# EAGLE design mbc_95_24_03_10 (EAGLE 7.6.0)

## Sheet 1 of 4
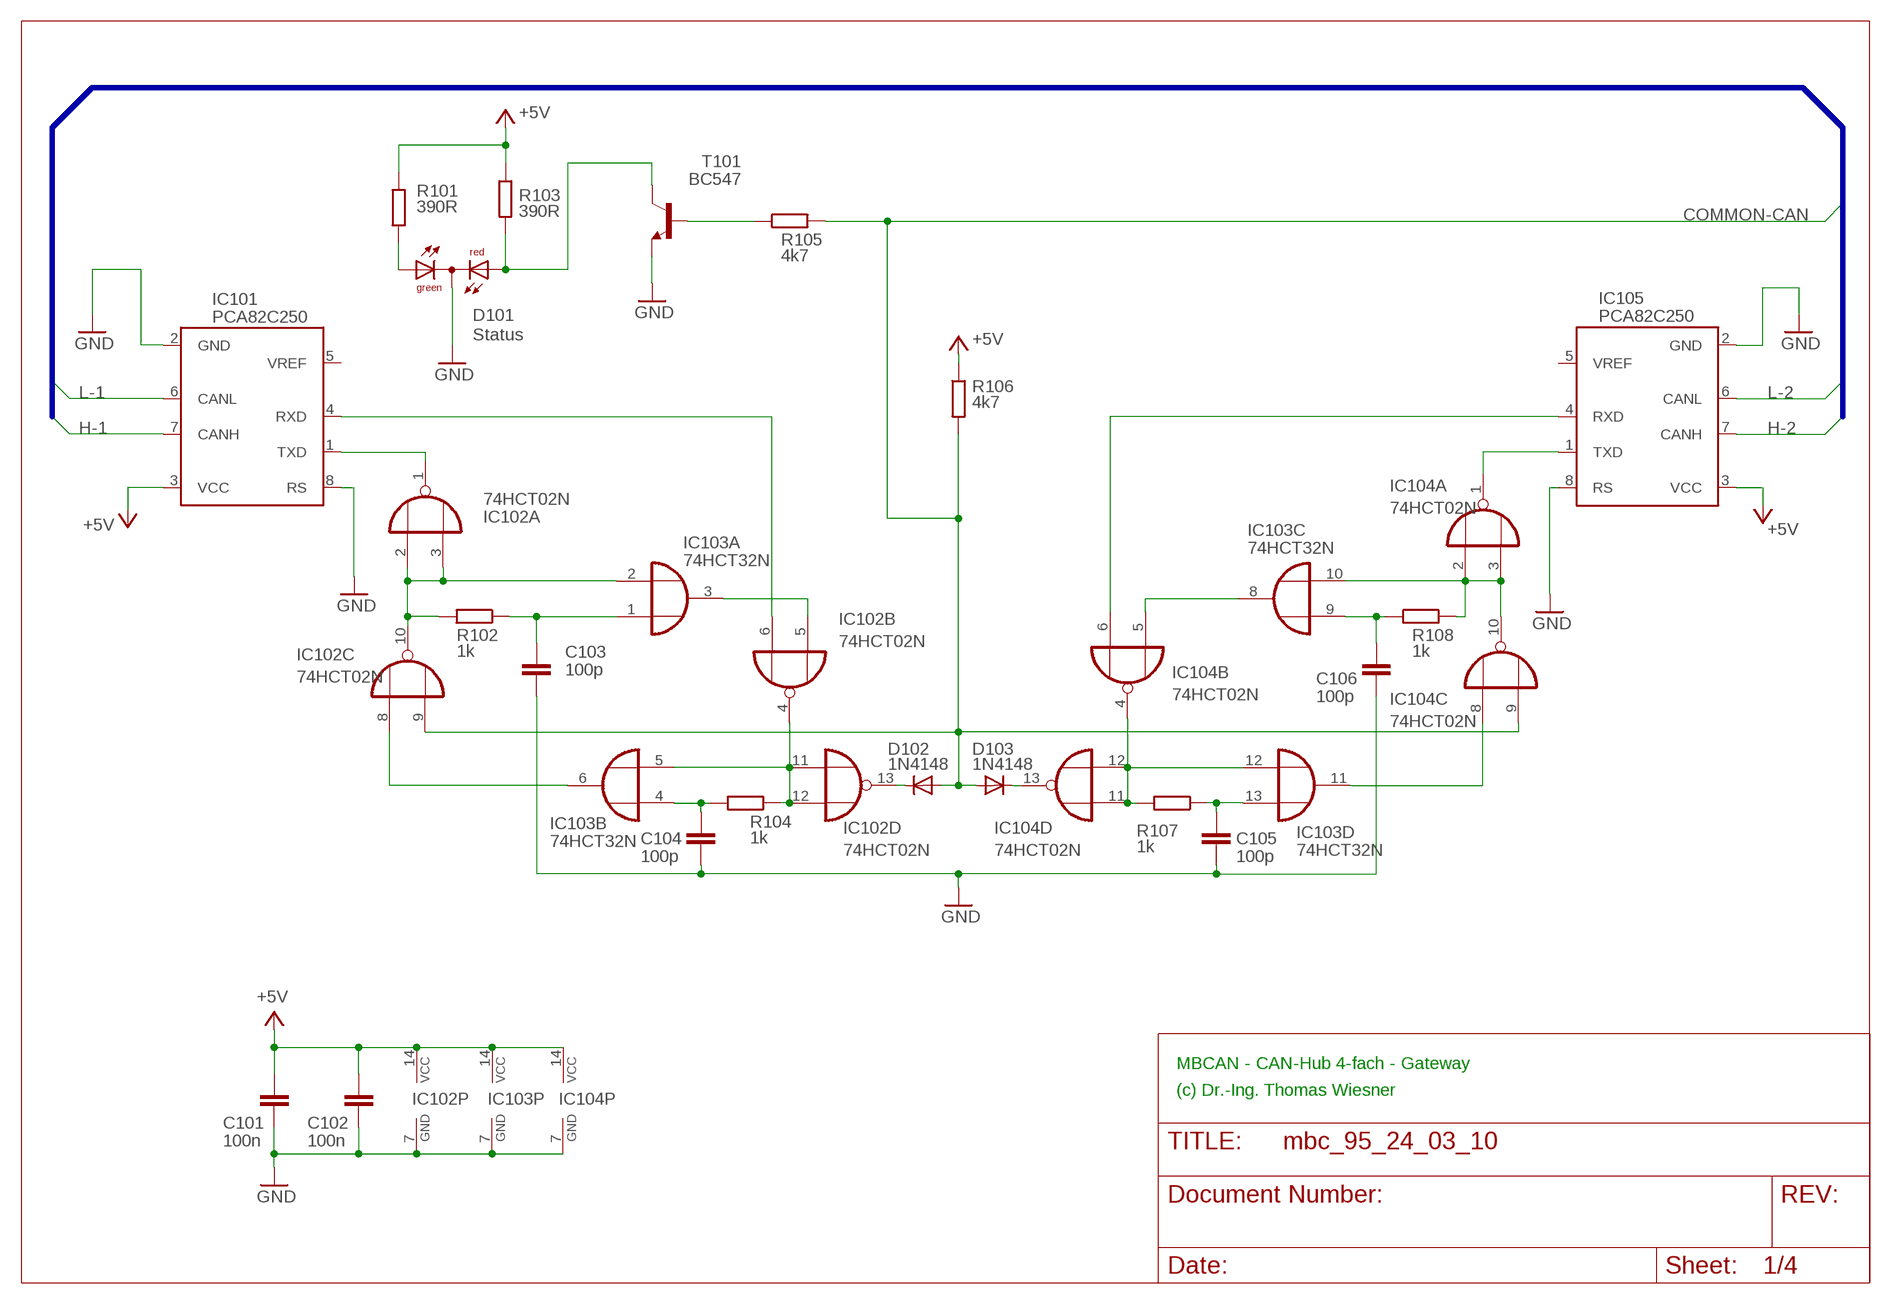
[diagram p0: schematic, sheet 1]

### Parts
C101  100n  C-EU025-025X050  [C025-025X050]
C102  100n  C-EU025-025X050  [C025-025X050]
C103  100p  C-EU025-025X050  [C025-025X050]
C104  100p  C-EU025-025X050  [C025-025X050]
C105  100p  C-EU025-025X050  [C025-025X050]
C106  100p  C-EU025-025X050  [C025-025X050]
D101  Status  DUOLED5MM  [DUOLED5MM]
D102  1N4148  1N4148DO35-10  [DO35-10]
D103  1N4148  1N4148DO35-10  [DO35-10]
IC101  PCA82C250  [DIL08]
IC102  74HCT02N  74HC02N  [DIL14]
IC103  74HCT32N  74HC32N  [DIL14]
IC104  74HCT02N  74HC02N  [DIL14]
IC105  PCA82C250  [DIL08]
R101  390R  R-EU_0207/10  [0207/10]
R102  1k  R-EU_0207/10  [0207/10]
R103  390R  R-EU_0207/10  [0207/10]
R104  1k  R-EU_0207/10  [0207/10]
R105  4k7  R-EU_0207/10  [0207/10]
R106  4k7  R-EU_0207/10  [0207/10]
R107  1k  R-EU_0207/10  [0207/10]
R108  1k  R-EU_0207/10  [0207/10]
T101  BC547  -NPN-TO92  [TO92]

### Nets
+5V: C101.2 C102.2 IC101.3(VCC) IC102.14(P:VCC) IC103.14(P:VCC) IC104.14(P:VCC) IC105.3(VCC) R101.1 R103.1 R106.1 ; also sheet 2,3,4
COMMON-CAN: D102.A D103.A IC102.9(C:I1) IC104.9(C:I1) R105.2 R106.2 ; also sheet 2,3
GND: C101.1 C102.1 C103.2 C104.2 C105.2 C106.2 D101.K(C) IC101.2(GND) IC101.8(RS) IC102.7(P:GND) IC103.7(P:GND) IC104.7(P:GND) IC105.2(GND) IC105.8(RS) T101.1(E) ; also sheet 2,3,4
H-1: IC101.7(CANH) ; also sheet 4
H-2: IC105.7(CANH) ; also sheet 4
L-1: IC101.6(CANL) ; also sheet 4
L-2: IC105.6(CANL) ; also sheet 4
N$1: IC102.2(A:I0) IC102.3(A:I1) IC102.10(C:O) IC103.2(A:I1) R102.2
N$2: R105.1 T101.2(B)
N$6: IC104.6(B:I1) IC105.4(RXD)
N$9: D101.AR R103.2 T101.3(C)
N$11: C103.1 IC103.1(A:I0) R102.1
N$13: D101.AG R101.2
N$14: IC101.1(TXD) IC102.1(A:O)
N$15: IC102.5(B:I0) IC103.3(A:O)
N$16: IC104.1(A:O) IC105.1(TXD)
N$17: IC102.8(C:I0) IC103.6(B:O)
N$18: C104.1 IC103.4(B:I0) R104.2
N$19: IC102.4(B:O) IC102.11(D:I0) IC102.12(D:I1) IC103.5(B:I1) R104.1
N$21: D102.C IC102.13(D:O)
N$25: IC101.4(RXD) IC102.6(B:I1)
N$27: D103.C IC104.13(D:O)
N$29: IC103.12(D:I0) IC104.4(B:O) IC104.11(D:I0) IC104.12(D:I1) R107.2
N$31: C105.1 IC103.13(D:I1) R107.1
N$33: IC103.11(D:O) IC104.8(C:I0)
N$34: IC103.10(C:I1) IC104.2(A:I0) IC104.3(A:I1) IC104.10(C:O) R108.1
N$36: C106.1 IC103.9(C:I0) R108.2
N$37: IC103.8(C:O) IC104.5(B:I0)
Unconnected: IC101.5(VREF) IC105.5(VREF)

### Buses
B$2

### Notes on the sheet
- MBCAN - CAN-Hub 4-fach - Gateway
- (c) Dr.-Ing. Thomas Wiesner

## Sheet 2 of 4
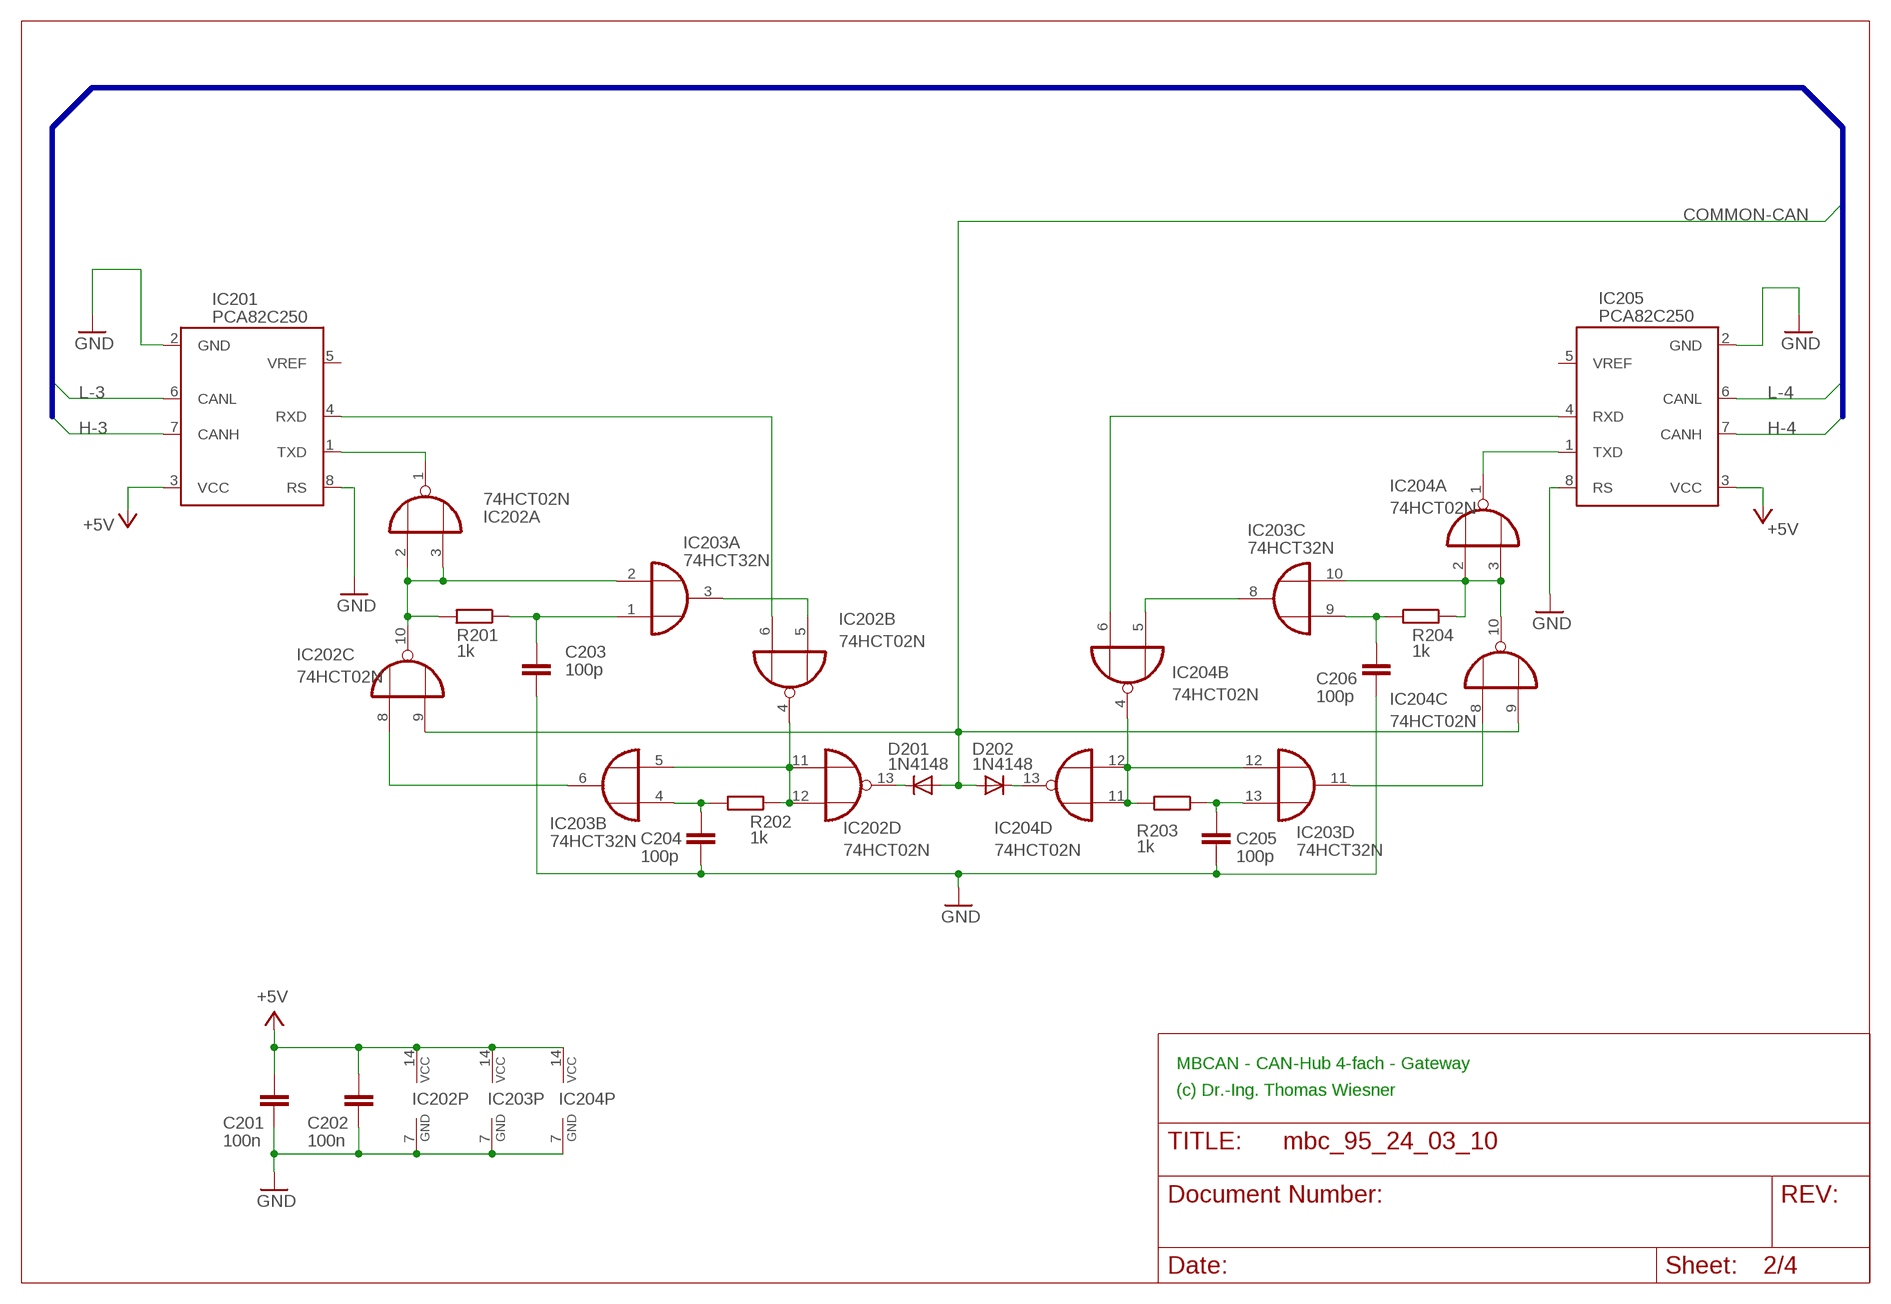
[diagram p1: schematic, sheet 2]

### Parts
C201  100n  C-EU025-025X050  [C025-025X050]
C202  100n  C-EU025-025X050  [C025-025X050]
C203  100p  C-EU025-025X050  [C025-025X050]
C204  100p  C-EU025-025X050  [C025-025X050]
C205  100p  C-EU025-025X050  [C025-025X050]
C206  100p  C-EU025-025X050  [C025-025X050]
D201  1N4148  1N4148DO35-10  [DO35-10]
D202  1N4148  1N4148DO35-10  [DO35-10]
IC201  PCA82C250  [DIL08]
IC202  74HCT02N  74HC02N  [DIL14]
IC203  74HCT32N  74HC32N  [DIL14]
IC204  74HCT02N  74HC02N  [DIL14]
IC205  PCA82C250  [DIL08]
R201  1k  R-EU_0207/10  [0207/10]
R202  1k  R-EU_0207/10  [0207/10]
R203  1k  R-EU_0207/10  [0207/10]
R204  1k  R-EU_0207/10  [0207/10]

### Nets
+5V: C201.2 C202.2 IC201.3(VCC) IC202.14(P:VCC) IC203.14(P:VCC) IC204.14(P:VCC) IC205.3(VCC) ; also sheet 1,3,4
COMMON-CAN: D201.A D202.A IC202.9(C:I1) IC204.9(C:I1) ; also sheet 1,3
GND: C201.1 C202.1 C203.2 C204.2 C205.2 C206.2 IC201.2(GND) IC201.8(RS) IC202.7(P:GND) IC203.7(P:GND) IC204.7(P:GND) IC205.2(GND) IC205.8(RS) ; also sheet 1,3,4
H-3: IC201.7(CANH) ; also sheet 4
H-4: IC205.7(CANH) ; also sheet 4
L-3: IC201.6(CANL) ; also sheet 4
L-4: IC205.6(CANL) ; also sheet 4
N$3: C203.1 IC203.1(A:I0) R201.1
N$23: IC202.5(B:I0) IC203.3(A:O)
N$24: IC202.8(C:I0) IC203.6(B:O)
N$26: C204.1 IC203.4(B:I0) R202.2
N$28: IC202.4(B:O) IC202.11(D:I0) IC202.12(D:I1) IC203.5(B:I1) R202.1
N$30: D201.C IC202.13(D:O)
N$32: D202.C IC204.13(D:O)
N$35: IC203.12(D:I0) IC204.4(B:O) IC204.11(D:I0) IC204.12(D:I1) R203.2
N$38: C205.1 IC203.13(D:I1) R203.1
N$39: IC203.11(D:O) IC204.8(C:I0)
N$41: IC203.10(C:I1) IC204.2(A:I0) IC204.3(A:I1) IC204.10(C:O) R204.1
N$43: C206.1 IC203.9(C:I0) R204.2
N$44: IC203.8(C:O) IC204.5(B:I0)
N$51: IC204.6(B:I1) IC205.4(RXD)
N$52: IC204.1(A:O) IC205.1(TXD)
N$53: IC201.4(RXD) IC202.6(B:I1)
N$54: IC201.1(TXD) IC202.1(A:O)
N$55: IC202.2(A:I0) IC202.3(A:I1) IC202.10(C:O) IC203.2(A:I1) R201.2
Unconnected: IC201.5(VREF) IC205.5(VREF)

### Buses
B$2

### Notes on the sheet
- MBCAN - CAN-Hub 4-fach - Gateway
- (c) Dr.-Ing. Thomas Wiesner

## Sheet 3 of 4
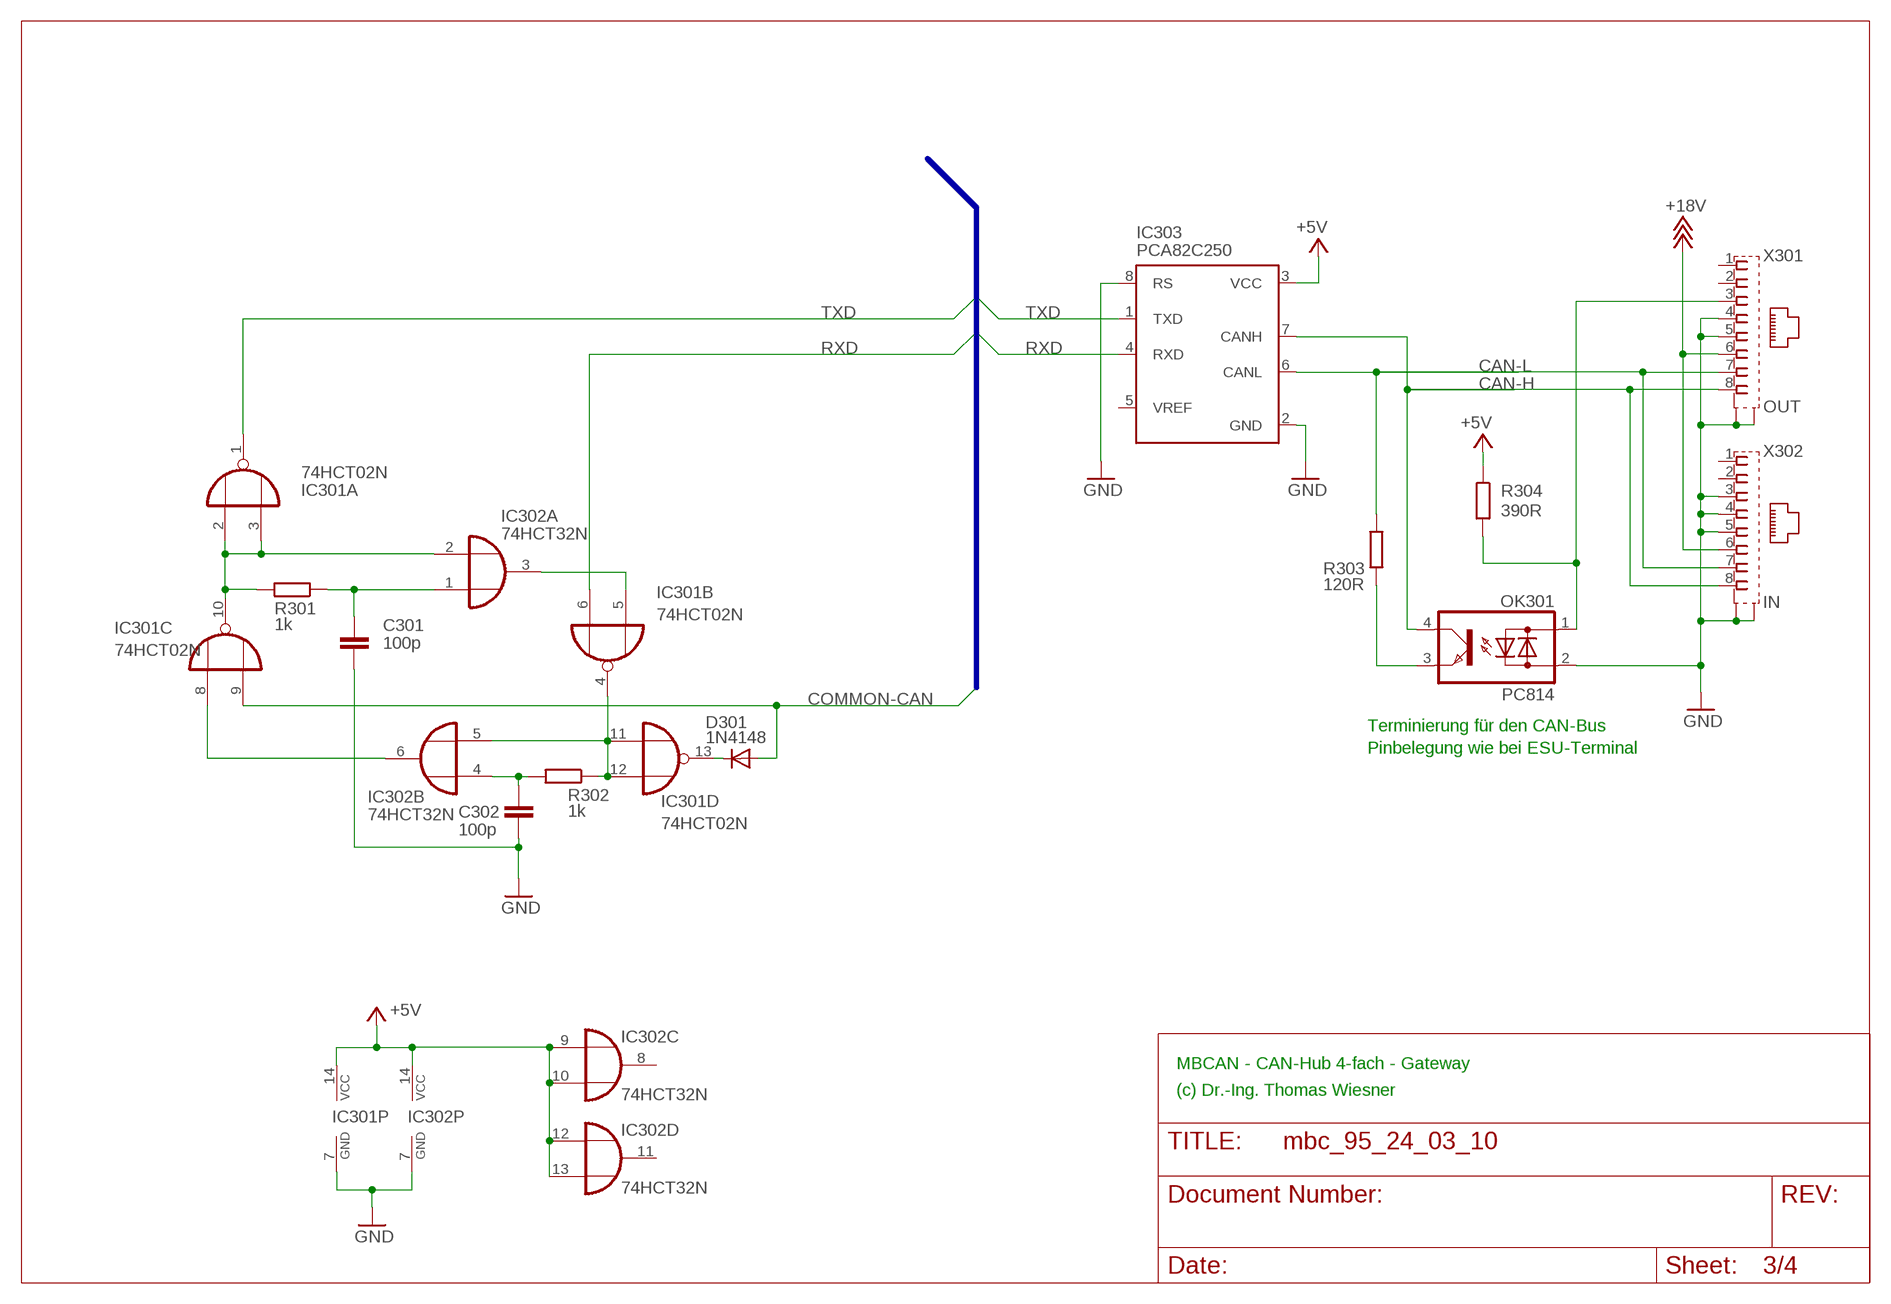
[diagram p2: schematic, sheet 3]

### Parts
C301  100p  C-EU025-025X050  [C025-025X050]
C302  100p  C-EU025-025X050  [C025-025X050]
D301  1N4148  1N4148DO35-10  [DO35-10]
IC301  74HCT02N  74HC02N  [DIL14]
IC302  74HCT32N  74HC32N  [DIL14]
IC303  PCA82C250  [DIL08]
OK301  PC814  [DIL04]
R301  1k  R-EU_0207/10  [0207/10]
R302  1k  R-EU_0207/10  [0207/10]
R303  120R  R-EU_0207/10  [0207/10]
R304  390R  R-EU_0207/10  [0207/10]
X301  OUT  0446200002  [0446200002]
X302  IN  0446200002  [0446200002]

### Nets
+5V: IC301.14(P:VCC) IC302.9(C:I0) IC302.10(C:I1) IC302.12(D:I0) IC302.13(D:I1) IC302.14(P:VCC) IC303.3(VCC) R304.1 ; also sheet 1,2,4
+18V: X301.6 X302.6 ; also sheet 4
CAN-H: IC303.7(CANH) OK301.4(C) X301.8 X302.8
CAN-L: IC303.6(CANL) R303.2 X301.7 X302.7
COMMON-CAN: D301.A IC301.9(C:I1) ; also sheet 1,2
GND: C301.2 C302.2 IC301.7(P:GND) IC302.7(P:GND) IC303.2(GND) IC303.8(RS) OK301.2(AC2) X301.4 X301.5 X301.S@1(S1) X301.S@2(S2) X302.3 X302.4 X302.5 X302.S@1(S1) X302.S@2(S2) ; also sheet 1,2,4
N$5: C301.1 IC302.1(A:I0) R301.1
N$7: IC301.5(B:I0) IC302.3(A:O)
N$8: IC301.8(C:I0) IC302.6(B:O)
N$10: C302.1 IC302.4(B:I0) R302.2
N$12: IC301.4(B:O) IC301.11(D:I0) IC301.12(D:I1) IC302.5(B:I1) R302.1
N$20: D301.C IC301.13(D:O)
N$42: OK301.3(E) R303.1
N$45: IC301.2(A:I0) IC301.3(A:I1) IC301.10(C:O) IC302.2(A:I1) R301.2
N$46: OK301.1(AC1) R304.2 X301.3
RXD: IC301.6(B:I1) IC303.4(RXD)
TXD: IC301.1(A:O) IC303.1(TXD)
Unconnected: IC302.8(C:O) IC302.11(D:O) IC303.5(VREF) X301.1 X301.2 X302.1 X302.2

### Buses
B$3

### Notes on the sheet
- Terminierung für den CAN-Bus
- Pinbelegung wie bei ESU-Terminal
- MBCAN - CAN-Hub 4-fach - Gateway
- (c) Dr.-Ing. Thomas Wiesner

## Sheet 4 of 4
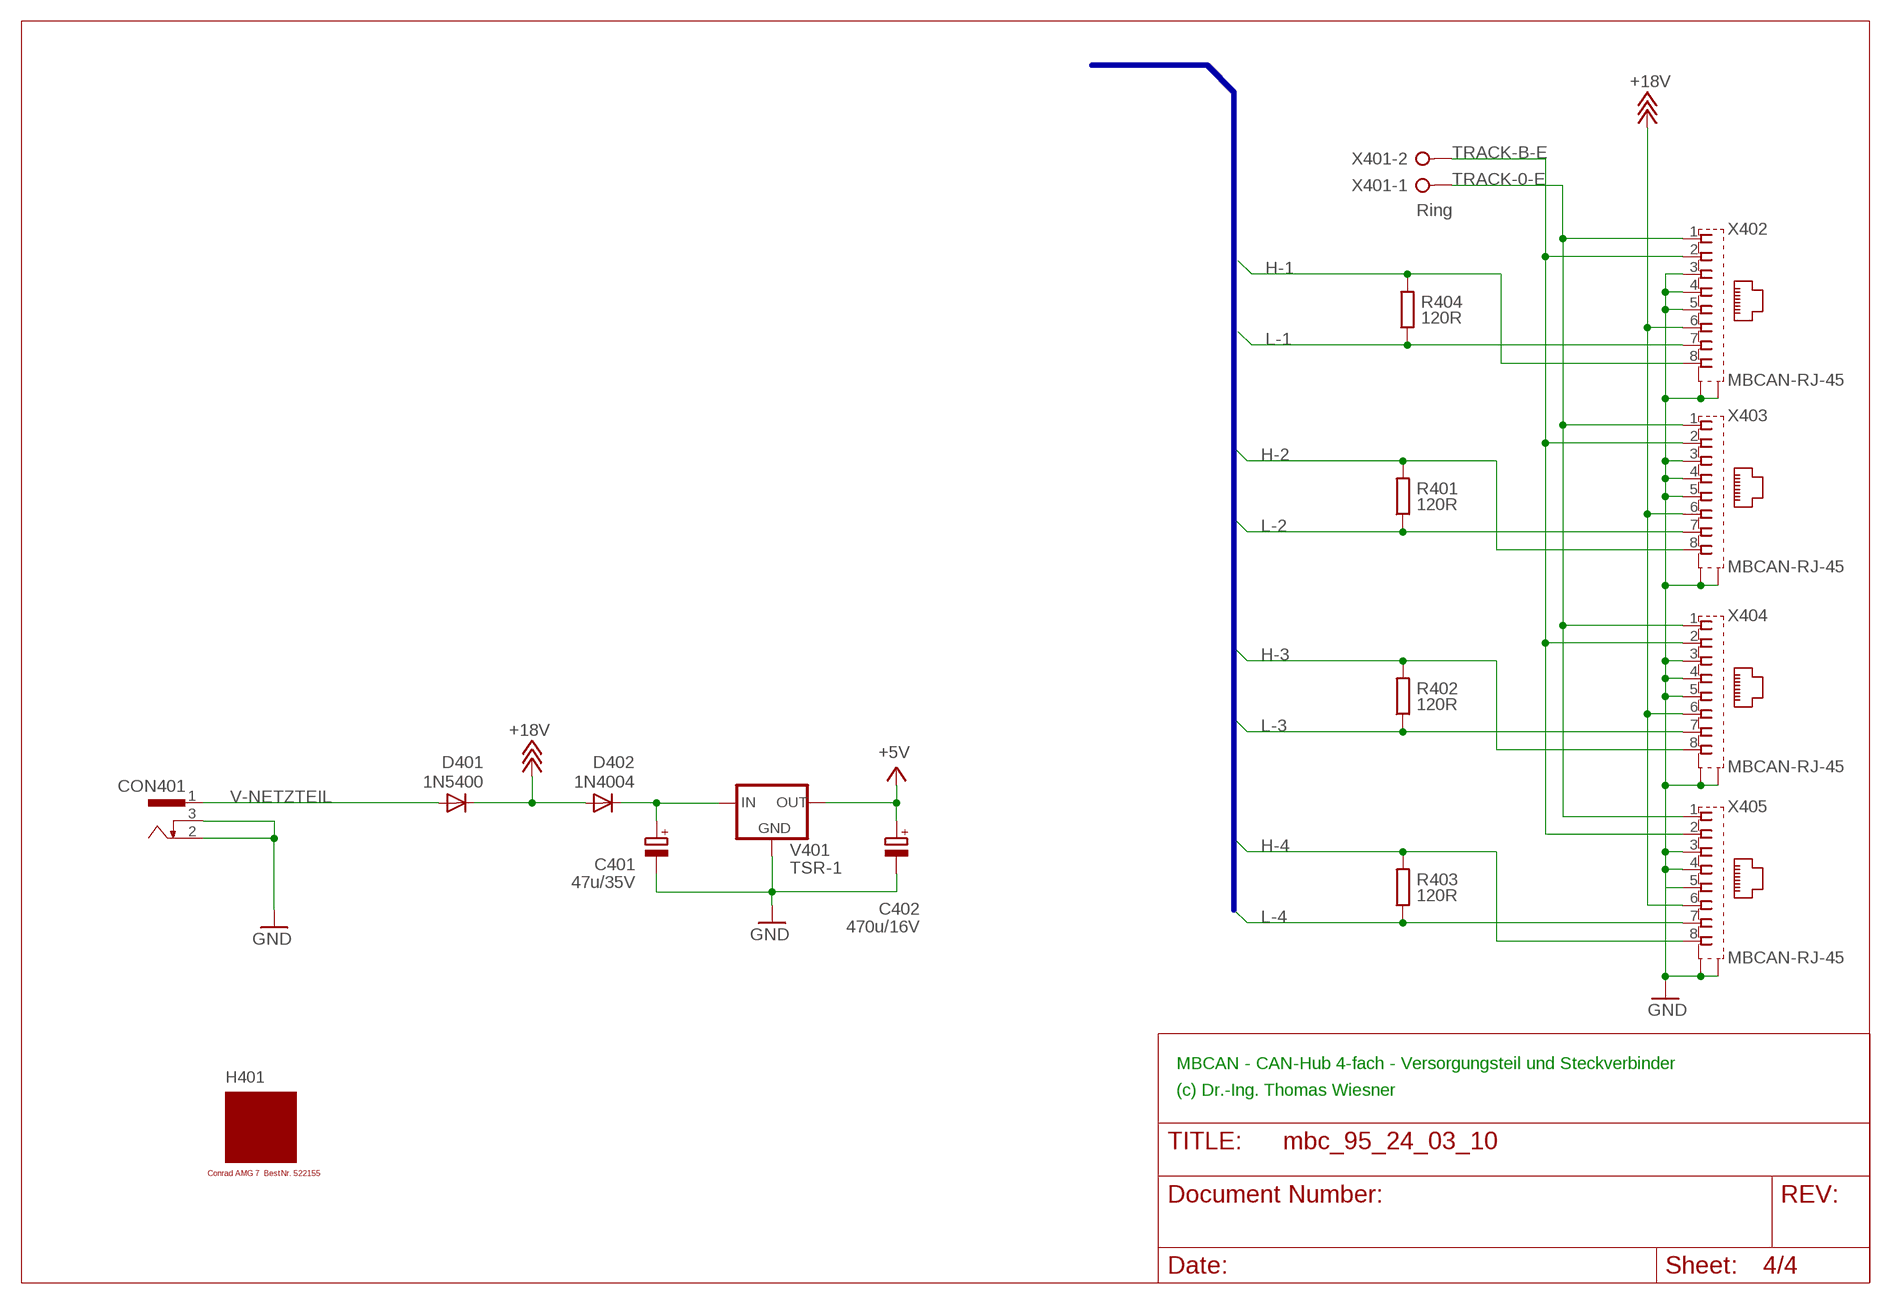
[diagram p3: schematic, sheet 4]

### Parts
C401  47u/35V  CPOL-EUE2.5-7  [E2,5-7]
C402  470u/16V  CPOL-EUE3.5-8  [E3,5-8]
CON401  POWER-JACK  [POWER-JACK]
D401  1N5400  [DO201-15]
D402  1N4004  [DO41-10]
H401  MODULGEHÄUSE-AMG-7  [MODULGEHÄUSE-AMG-7]
R401  120R  R-EU_0207/10  [0207/10]
R402  120R  R-EU_0207/10  [0207/10]
R403  120R  R-EU_0207/10  [0207/10]
R404  120R  R-EU_0207/10  [0207/10]
V401  TSR-1  [TRACO-TSR-1]
X401  Ring  W237-02P  [W237-132]
X402  MBCAN-RJ-45  [0446200002]
X403  MBCAN-RJ-45  [0446200002]
X404  MBCAN-RJ-45  [0446200002]
X405  MBCAN-RJ-45  [0446200002]

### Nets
+5V: C402.+ V401.OUT ; also sheet 1,2,3
+18V: D401.C D402.A X402.6 X403.6 X404.6 X405.6 ; also sheet 3
GND: C401.- C402.- CON401.2 CON401.3 V401.GND X402.3 X402.4 X402.5 X402.S@1(S1) X402.S@2(S2) X403.3 X403.4 X403.5 X403.S@1(S1) X403.S@2(S2) X404.3 X404.4 X404.5 X404.S@1(S1) X404.S@2(S2) X405.3 X405.4 X405.5 X405.S@1(S1) X405.S@2(S2) ; also sheet 1,2,3
H-1: R404.2 X402.8 ; also sheet 1
H-2: R401.2 X403.8 ; also sheet 1
H-3: R402.2 X404.8 ; also sheet 2
H-4: R403.2 X405.8 ; also sheet 2
L-1: R404.1 X402.7 ; also sheet 1
L-2: R401.1 X403.7 ; also sheet 1
L-3: R402.1 X404.7 ; also sheet 2
L-4: R403.1 X405.7 ; also sheet 2
N$4: C401.+ D402.C V401.IN
TRACK-0-E: X401.1 X402.1 X403.1 X404.1 X405.1
TRACK-B-E: X401.2 X402.2 X403.2 X404.2 X405.2
V-NETZTEIL: CON401.1 D401.A

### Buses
B$1

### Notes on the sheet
- MBCAN - CAN-Hub 4-fach - Versorgungsteil und Steckverbinder
- (c) Dr.-Ing. Thomas Wiesner

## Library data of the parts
C101-C106 C201-C206 C301 C302 = rcl:C-EU: CAPACITOR, European symbol
C401 C402 = rcl:CPOL-EU: POLARIZED CAPACITOR, European symbol
CON401 = mbc:POWER-JACK: Power-Stecker für 2,5 mm Hohlbuchse
D101 = led:DUOLED5MM: DUO LED 2 colors, 5 mm, round
D102 D103 D201 D202 D301 = diode:1N4148: DIODE
D401 = diode:1N5400: DIODE
D402 = diode:1N4004: DIODE
H401 = mbc:MODULGEHÄUSE-AMG-7: Gehäuse
IC101 IC105 IC201 IC205 IC303 = micro-philips:PCA82C250: CAN CONTROLLER INTERFACE; OC_FARNELL: 3692358; OC_NEWARK: unknown
IC102 IC104 IC202 IC204 IC301 = 74xx-eu:74*02: Quad 2-input NOR gate
IC103 IC203 IC302 = 74xx-eu:74*32: Quad 2-input OR gate
OK301 = optocoupler:PC814: SHARP OPTO COUPLER; OC_FARNELL: 9707662; OC_NEWARK: unknown
R101-R108 R201-R204 R301-R304 R401-R404 = resistor:R-EU_: RESISTOR, European symbol
T101 = transistor:*-NPN-: NPN Transistror BF959 corrected 2008.03.06
V401 = mbc:TSR-1: Spannungsregler Hersteller: TRACO Typ: TSR-1 5V: TSR 1-2450 Spg: 5V Strom: 1A Reichelt TSR 1-2450
X301 X302 = mbc:0446200002: RJ-45 INVERTED MODULAR JACK ASSEMBLY WITH RJ-11 KEEPOUT FEATURE Source: Data sheet MOLEX 0446200002 BUCHSE, RJ45, GESCHIRMT Source: Farnell; MF: MOLEX; MPN: 0446200002; OC_FARNELL: 9251910
X401 = con-wago-508:W237-02P: WAGO SREW CLAMP; OC_FARNELL: unknown; OC_NEWARK: unknown
X402-X405 = mbc:MBCAN-RJ-45: RJ-45 INVERTED MODULAR JACK ASSEMBLY WITH RJ-11 KEEPOUT FEATURE Source: Data sheet MOLEX 0446200002 BUCHSE, RJ45, GESCHIRMT Source: Farnell; MF: MOLEX; MPN: 0446200002; OC_FARNELL: 9251910

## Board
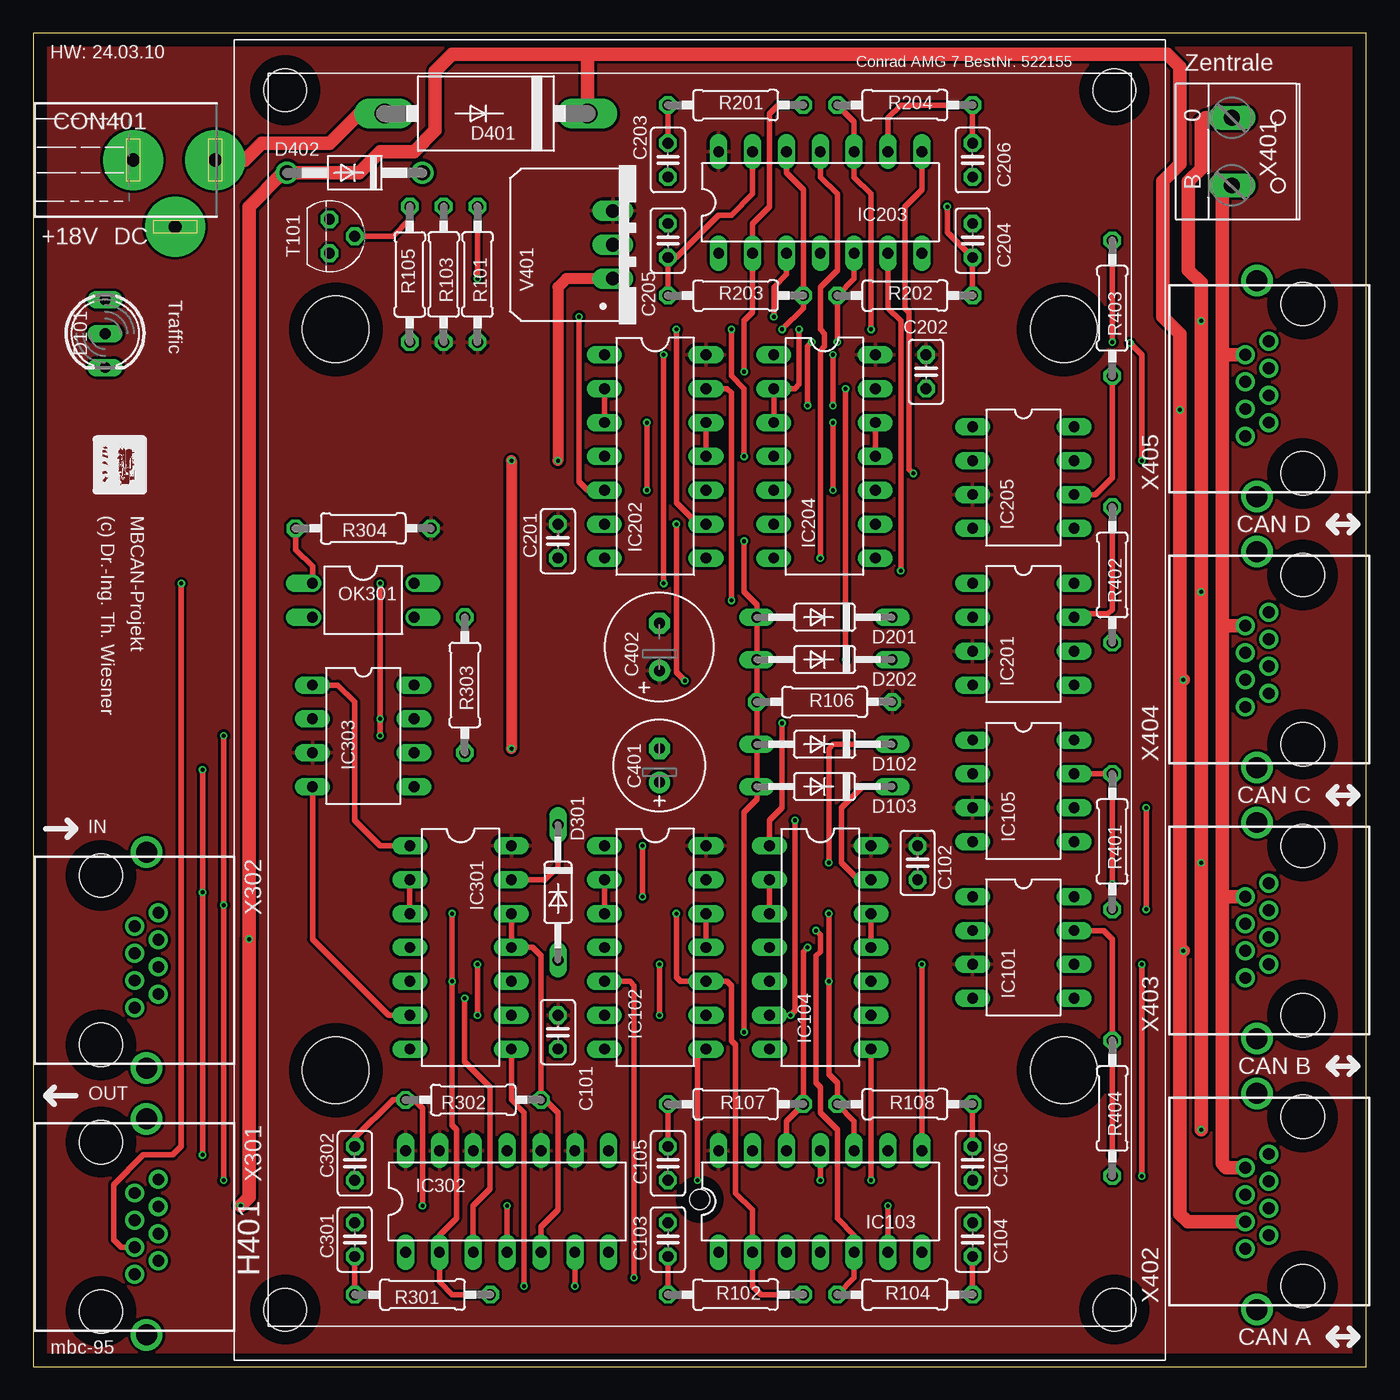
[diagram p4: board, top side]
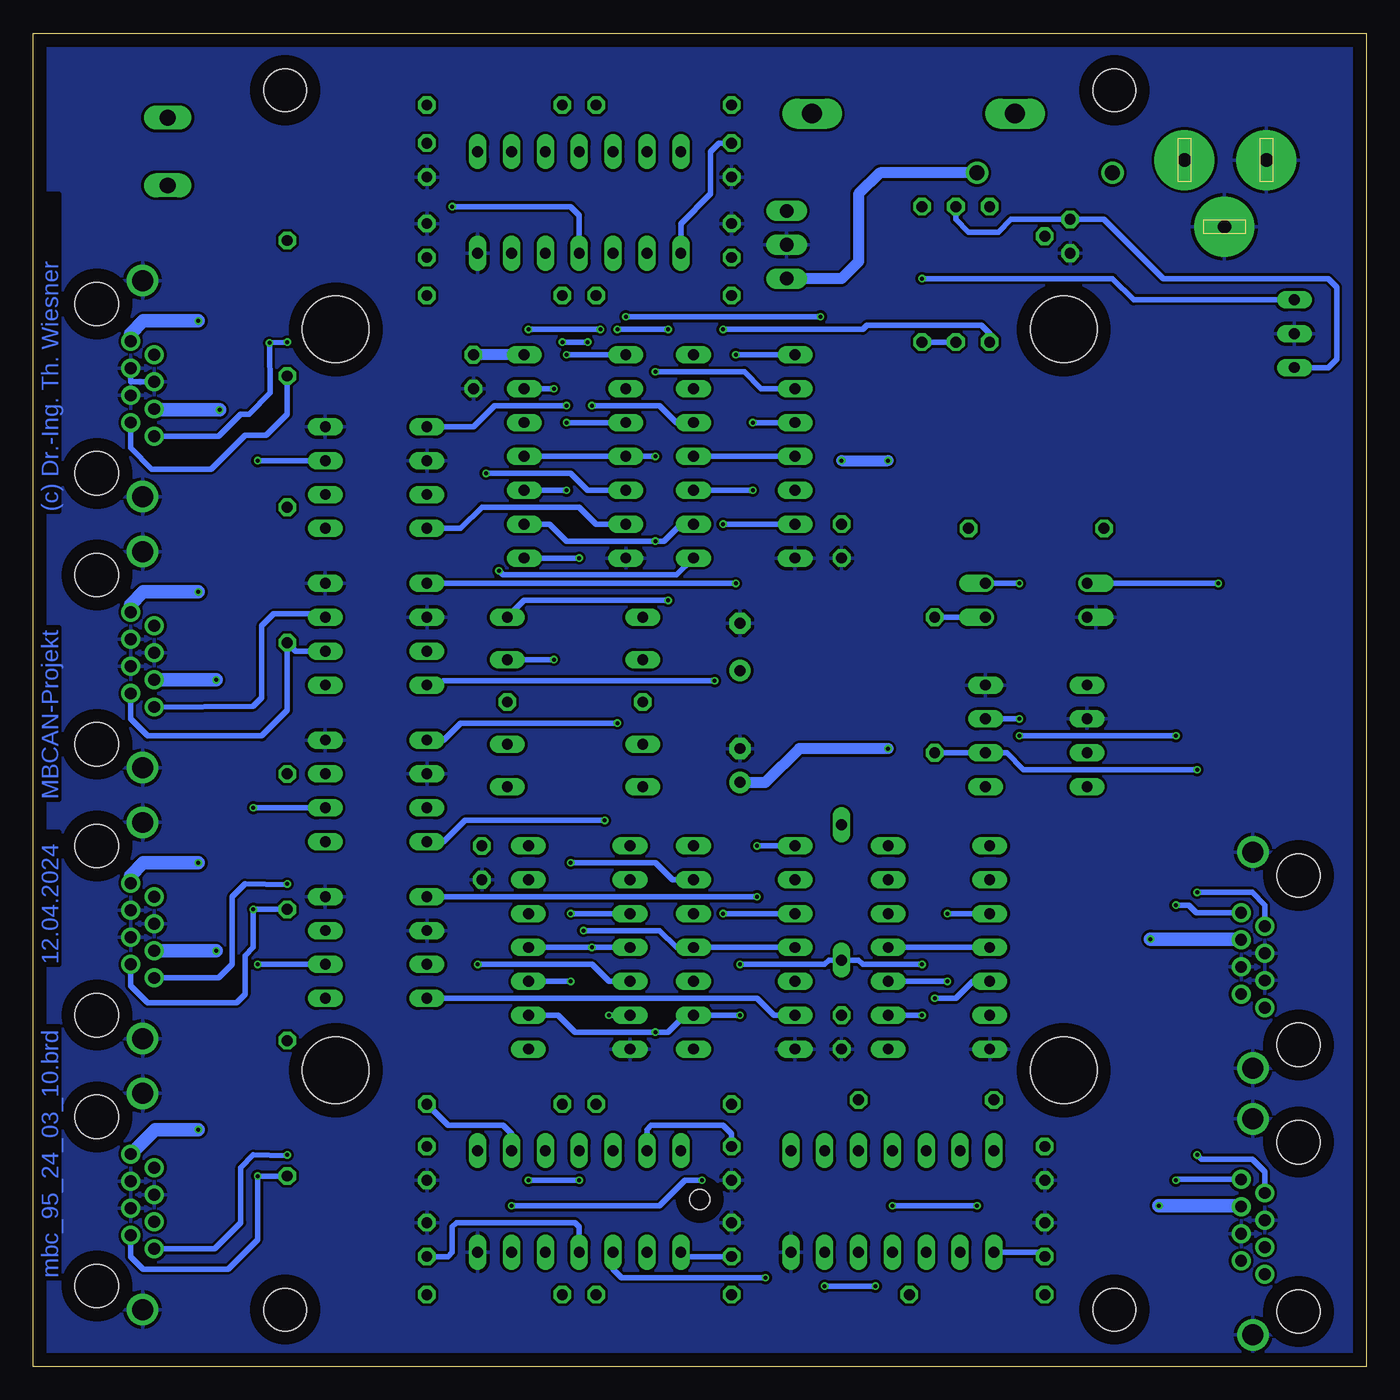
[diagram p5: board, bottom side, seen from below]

Size 100 x 99.99 mm. Coordinates in mm from the lower left corner, seen from the top.
Outline: 100,0 100,99.99 0,99.99 0,0 100,0
Copper layers (1*16): Top 0.035mm / dielectric 1.5mm / Bottom 0.035mm
Design rules "default *": minimum track width 10mil, minimum drill 0.00761875mm, track to track 8mil, track to pad 8mil, pad to pad 8mil, via to via 8mil, smd to smd 8mil, copper to edge 40mil, drill to drill 8mil, minimum pad ring 10mil, minimum via ring 0.125mm, stop-mask expansion 4mil, vias tented up to drill 0mil, thermal gap 10mil

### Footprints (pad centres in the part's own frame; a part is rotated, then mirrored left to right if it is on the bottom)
C025-025X050 = drill 0.813 octagon: 1 -1.27,0; 2 1.27,0
E2,5-7 = drill 0.813 pad 1.6: + -1.27,0 | drill 0.813 pad 1.6 octagon: - 1.27,0
E3,5-8 = drill 0.813 pad 1.6: + -1.778,0 | drill 0.813 pad 1.6 octagon: - 1.778,0
POWER-JACK = drill 1 pad 4.5: 1 0,6.03; 2 0,-0.12; 3 5,3.03
DUOLED5MM = drill 0.813 long: AG -2.54,0; AR 2.54,0; K 0,0
DO35-10 = drill 0.813 long: A 5.08,0; C -5.08,0
DO201-15 = drill 1.499 long: A 7.62,0; C -7.62,0
DO41-10 = drill 1.118: A 5.08,0; C -5.08,0
MODULGEHÄUSE-AMG-7 = hole 3.2: -45.72,-31.115; -45.72,31.115; 45.72,31.115; 45.72,-31.115 | hole 5: -27.781,-27.305; 27.781,-27.305; -27.781,27.305; 27.781,27.305 | hole 1.5: -37.465,0
DIL08 = drill 0.813 long: 1 -3.81,-3.81; 2 -1.27,-3.81; 3 1.27,-3.81; 4 3.81,-3.81; 5 3.81,3.81; 6 1.27,3.81; 7 -1.27,3.81; 8 -3.81,3.81
DIL14 = drill 0.813 long: 1 -7.62,-3.81; 2 -5.08,-3.81; 3 -2.54,-3.81; 4 0,-3.81; 5 2.54,-3.81; 6 5.08,-3.81; 7 7.62,-3.81; 8 7.62,3.81; 9 5.08,3.81; 10 2.54,3.81; 11 0,3.81; 12 -2.54,3.81; 13 -5.08,3.81; 14 -7.62,3.81
DIL04 = drill 0.813 offset: 1 -1.27,-3.81; 2 1.27,-3.81; 3 1.27,3.81; 4 -1.27,3.81
0207/10 = drill 0.813 octagon: 1 -5.08,0; 2 5.08,0
TO92 = drill 0.813 octagon: 1 1.27,0; 2 0,1.905; 3 -1.27,0
TRACO-TSR-1 = drill 1.016 long: GND 0,2.54; IN -2.54,2.54; OUT 2.54,2.54
0446200002 = drill 0.889 pad 1.422: 1 3.556,2.54; 2 2.54,4.318; 3 1.524,2.54; 4 0.508,4.318; 5 -0.508,2.54; 6 -1.524,4.318; 7 -2.54,2.54; 8 -3.556,4.318 | drill 1.575 pad 2.286: S@1 -8.103,3.429; S@2 8.103,3.429 | hole 3.251: 6.35,0; -6.35,0
W237-132 = drill 1.194 long: 1 -2.54,-0.635; 2 2.54,-0.635

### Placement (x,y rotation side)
C101  39.36,25.08 90 top
C102  66.34,37.78 90 top
C103  47.61,9.53 90 top
C104  70.47,9.53 90 top
C105  47.61,15.24 270 top
C106  70.47,15.24 270 top
C201  39.36,61.91 90 top
C202  66.98,74.61 90 top
C203  47.61,90.49 270 top
C204  70.47,84.45 90 top
C205  47.61,84.45 90 top
C206  70.47,90.49 270 top
C301  24.12,9.53 90 top
C302  24.12,15.24 270 top
C401  46.98,45.09 90 top
C402  46.98,53.98 90 top
CON401  7.61,90.49 270 top
D101  5.38,77.47 270 top
D102  59.36,46.67 180 top
D103  59.36,43.5 180 top
D201  59.36,56.2 180 top
D202  59.36,53.02 180 top
D301  39.36,35.56 270 top
D401  33.96,93.98 180 top
D402  24.12,89.53 180 top
H401  50,50 90 top
IC101  74.28,31.43 270 top
IC102  46.66,31.43 270 top
IC103  59.04,12.38 0 top
IC104  59.04,31.43 270 top
IC105  74.28,43.18 270 top
IC201  74.28,54.93 270 top
IC202  46.66,68.26 270 top
IC203  59.04,87.31 0 top
IC204  59.36,68.26 270 top
IC205  74.28,66.67 270 top
IC301  32.05,31.43 270 top
IC302  35.55,12.38 0 top
IC303  24.75,47.31 270 top
OK301  24.75,57.47 270 top
R101  33.32,81.92 90 top
R102  52.69,5.4 0 top
R103  30.79,81.92 90 top
R104  65.39,5.4 0 top
R105  28.25,81.92 270 top
R106  59.36,49.85 180 top
R107  52.69,19.68 0 top
R108  65.39,19.68 0 top
R201  52.69,94.61 0 top
R202  65.39,80.33 0 top
R203  52.69,80.33 0 top
R204  65.39,94.61 0 top
R301  29.2,5.4 0 top
R302  33.01,20 180 top
R303  32.37,51.12 270 top
R304  24.75,62.87 180 top
R401  80.95,39.37 90 top
R402  80.95,59.37 90 top
R403  80.95,79.38 90 top
R404  80.95,19.37 90 top
T101  22.21,84.77 270 top
V401  46.02,84.14 90 top
X301  5.07,10.48 270 top
X302  5.07,30.48 270 top
X401  90.55,91.12 270 top
X402  95.24,12.38 90 top
X403  95.24,32.7 90 top
X404  95.24,53.02 90 top
X405  95.24,73.34 90 top

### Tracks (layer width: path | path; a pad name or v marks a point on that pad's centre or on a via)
+5V
  Bottom 0.406: R101.1 R103.1
  Bottom 0.813: IC204.14 C202.2
  pour Top: -0.01,100.01 100,100.01 100,0 -0.01,0
+18V  (via drill 0.3)
  Top 1.016: X402.6 86.6,10.86 86.03,11.43 86.03,31.43 | 86.03,31.43 86.03,51.75 | 86.03,51.75 v86.03,71.75 86.03,77.47 84.76,78.74 84.76,88.9 86.03,90.17 86.03,97.47 85.08,98.42 41.58,98.42 | v86.28,51.5 86.03,51.75 | v86.28,31.18 86.03,31.43 | 41.58,98.42 31.42,98.42 30.15,97.16 30.15,92.71 28.56,91.12 26.02,91.12 24.44,89.53 D402.A 18.72,89.53 16.18,87 v16.18,32.07 16.18,12.7 v15.54,12.06 | 41.58,98.42 D401.C
  Bottom 1.016: v86.03,71.75 90.86,71.75 X405.6 | X404.6 v86.28,51.5 | X403.6 v86.28,31.18 | X301.6 9.45,12.06 v15.54,12.06 | v16.18,32.07 9.45,32.07 X302.6
CAN-H  (via drill 0.3)
  Top 0.406: v14.27,13.97 v14.27,34.61 v14.27,47.31 | v26.02,47.31 v26.02,48.58 v26.02,58.74
  Bottom 0.406: X301.8 14.21,14.03 v14.27,13.97 | v14.27,47.31 v26.02,47.31 | v26.02,58.74 OK301.4 | IC303.7 v26.02,48.58 | X302.8 12.75,34.04 13.32,34.61 v14.27,34.61
CAN-L  (via drill 0.3)
  Top 0.406: v12.69,44.77 v12.69,35.56 v12.69,15.88
  Bottom 0.406: X302.7 7.61,34.61 8.56,35.56 v12.69,35.56 | v12.69,44.77 25.71,44.77 26.98,46.04 IC303.6 R303.2 | X301.7 7.61,14.61 8.56,15.56 12.37,15.56 v12.69,15.88
COMMON-CAN  (via drill 0.3)
  Top 0.406: v53.33,61.91 53.33,58.1 54.28,57.15 D201.A D202.A R106.2 D102.A D103.A 54.28,42.55 53.33,41.59 v53.33,25.08 | v33.32,30.16 v33.32,26.35 | v46.98,30.16 v46.98,26.35 | v48.25,77.79 48.25,64.77 49.52,63.5 50.15,63.5 IC202.9
  Bottom 0.406: IC204.9 61.27,63.18 60,61.91 v53.33,61.91 52.69,61.91 51.42,63.18 IC202.9 | IC104.9 60.63,26.35 59.36,25.08 v53.33,25.08 52.38,25.08 51.1,26.35 IC102.9 v46.98,26.35 | v33.32,30.16 37.77,30.16 38.09,30.48 D301.A 40.31,30.48 40.63,30.16 v46.98,30.16 | v33.32,26.35 IC301.9 | R105.2 28.25,77.47 28.88,78.11 37.45,78.11 37.77,77.79 v48.25,77.79
GND
  Bottom 0.406: X405.4 92.7,73.85 X405.3
  pour Bottom: -0.01,100.01 100,100.01 100,0 -0.01,0
H-1  (via drill 0.3)
  Top 0.406: v80.95,15.88 R404.2 80.95,32.07 80.32,32.7 IC101.7
  Bottom 0.406: X402.8 86.41,8.83 84.44,10.79 84.44,14.92 83.49,15.88 81.01,15.81 v80.95,15.88
H-2  (via drill 0.3)
  Top 0.406: v80.95,36.2 R401.2 IC105.7
  Bottom 0.406: X403.8 86.09,29.15 85.08,30.16 85.08,35.24 84.13,36.2 81.01,36.13 v80.95,36.2
H-3
  Top 0.406: R402.2 80.95,56.77 80.63,56.45 78.35,56.45 IC201.7
  Bottom 0.406: X404.8 83.49,49.53 82.86,50.16 82.86,55.56 81.97,56.45 79.3,56.45 79.05,56.2 IC201.7
H-4  (via drill 0.3)
  Top 0.406: v80.95,76.83 R403.2 | v82.28,76.77 83.17,75.88 v83.17,67.94
  Bottom 0.406: X405.8 86.09,69.79 84.44,71.44 83.81,71.44 82.22,73.03 v82.28,76.77 v80.95,76.83 | v83.17,67.94 IC205.7
L-1  (via drill 0.3)
  Top 0.406: v83.17,30.16 v83.17,14.29
  Bottom 0.406: R404.1 v83.17,14.29 83.17,9.53 85.39,7.3 91.74,7.3 92.7,8.26 X402.7 | IC101.6 v83.17,30.16
L-2  (via drill 0.3)
  Top 0.406: v83.49,41.91 v83.49,34.29
  Bottom 0.406: R401.1 v83.49,34.29 83.49,31.43 84.13,30.8 84.13,27.94 84.76,27.3 91.43,27.3 92.7,28.57 X403.7 | IC105.6 v83.49,41.91
L-3
  Bottom 0.406: X404.7 92.7,48.58 91.43,47.31 82.86,47.31 80.95,49.21 R402.1 80.32,53.66 IC201.6
L-4
  Top 0.406: R403.1 80.95,66.67 79.68,65.41 IC205.6
  Bottom 0.406: R403.1 80.95,71.44 82.54,69.85 84.13,69.85 86.66,67.31 91.11,67.31 92.7,68.9 X405.7
N$1  (via drill 0.3)
  Top 0.406: IC102.2 IC102.3 | v48.25,33.97 48.25,29.21 48.57,28.89 IC102.10 52.06,28.89 52.38,28.57 52.38,24.45 52.69,24.13 52.69,13.02 53.96,11.75 IC103.2 53.96,6.03 54.6,5.4 R102.2
  Bottom 0.406: v48.25,33.97 IC102.3
N$2
  Top 0.406: T101.2 26.98,84.77 28.25,86.04 R105.1
N$3
  Top 0.406: R201.1 C203.1
  Bottom 0.406: C203.1 48.57,91.76 49.2,91.12 49.2,87.95 51.42,85.72 IC203.1
N$4  (via drill 0.3)
  Top 0.813: V401.IN 39.99,81.6 39.36,80.96 v39.36,67.94 | v35.86,67.94 v35.86,46.35
  Bottom 0.813: C401.+ 45.07,43.81 42.53,46.35 v35.86,46.35 | D402.C 36.5,89.53 38.09,87.95 38.09,82.87 39.36,81.6 V401.IN | v39.36,67.94 v35.86,67.94
N$5
  Top 0.406: R301.1 C301.1
  Bottom 0.406: IC302.1 24.44,8.57 C301.1
N$6  (via drill 0.3)
  Top 0.406: v56.82,26.35 57.14,26.67 v57.14,40.96
  Bottom 0.406: IC104.6 v56.82,26.35 | v57.14,40.96 67.61,40.96 69.2,39.37 IC105.4
N$7  (via drill 0.3)
  Top 0.406: IC302.3 33.01,12.06 34.28,13.34 34.28,20.95 32.37,22.86 v32.37,27.62
  Bottom 0.406: v32.37,27.62 30.78,27.62 29.51,28.89 IC301.5
N$8  (via drill 0.3)
  Top 0.406: IC301.8 35.86,20 36.82,19.05 v36.82,6.03 | v40.63,6.03 IC302.6
  Bottom 0.406: v36.82,6.03 v40.63,6.03
N$9
  Bottom 0.406: D101.AR 2.84,74.93 2.21,75.56 2.21,80.96 2.84,81.6 15.23,81.6 19.67,86.04 T101.3 26.66,86.04 27.61,85.09 29.83,85.09 30.78,86.04 R103.2
N$10  (via drill 0.3)
  Top 0.406: C302.1 24.12,17.14 26.98,20 R302.2 28.56,20 29.2,19.37 v29.2,12.06 | v35.55,12.06 IC302.4
  Bottom 0.406: v29.2,12.06 v35.55,12.06
N$11
  Top 0.406: R102.1 C103.1
  Bottom 0.406: C103.1 51.1,8.26 IC103.1
N$12
  Top 0.406: IC301.12 IC301.11 37.45,31.43 38.09,30.8 R302.1 38.4,20 39.36,19.05 39.36,11.75 38.09,10.48 IC302.5
  Bottom 0.406: IC301.4 IC301.11
N$13  (via drill 0.3)
  Top 0.406: v33.32,81.6 R101.2
  Bottom 0.406: D101.AG 17.45,80.01 19.04,81.6 v33.32,81.6
N$14  (via drill 0.3)
  Top 0.406: v45.71,35.24 v45.71,39.05
  Bottom 0.406: IC101.1 v45.71,35.24 | v45.71,39.05 IC102.1
N$15  (via drill 0.3)
  Top 0.406: IC102.5 44.75,28.89 45.07,28.57 v45.07,6.67
  Bottom 0.406: v45.07,6.67 55.87,6.67 56.5,7.3 IC103.3
N$16  (via drill 0.3)
  Top 0.406: IC104.1 55.23,40.96 56.18,41.91 v56.18,48.26
  Bottom 0.406: v56.18,48.26 67.93,48.26 69.2,46.99 IC105.1
N$17  (via drill 0.3)
  Top 0.406: IC103.6 v64.12,12.06 | v49.83,13.97 49.83,23.18 IC102.8
  Bottom 0.406: v64.12,12.06 53.01,12.06 51.1,13.97 v49.83,13.97
N$18
  Top 0.406: R104.2 C104.1
  Bottom 0.406: IC103.4 59.04,10.48 59.36,10.79 68.25,10.79 68.57,10.48 68.57,8.57 68.88,8.26 C104.1
N$19  (via drill 0.3)
  Top 0.406: IC102.12 IC102.11 | v58.72,32.7 59.04,32.38 59.04,31.11 58.72,30.8 58.72,21.27 59.04,20.95 59.04,19.05 60.31,17.78 60.31,11.11 61.58,9.84 IC103.5 61.58,6.67 R104.1
  Bottom 0.406: IC102.4 IC102.11 51.74,31.43 53.01,32.7 v58.72,32.7
N$20
  Top 0.406: D301.C 39.36,37.47 38.4,36.51 IC301.13
N$21  (via drill 0.3)
  Top 0.406: D102.C 60,46.67 59.68,46.35 v59.68,37.78
  Bottom 0.406: v59.68,37.78 53.33,37.78 52.06,36.51 IC102.13
N$23  (via drill 0.3)
  Top 0.406: IC203.3 56.5,81.92 55.55,80.96 v55.55,78.74 | v40.95,78.74 40.95,66.36 41.58,65.72 IC202.5
  Bottom 0.406: v55.55,78.74 v40.95,78.74
N$24  (via drill 0.3)
  Top 0.406: IC203.6 64.12,79.38 65.08,78.42 v65.08,59.69
  Bottom 0.406: v65.08,59.69 64.76,59.37 51.74,59.37 IC202.8
N$25
  Bottom 0.406: IC101.4 45.71,27.62 44.44,26.35 IC102.6
N$26  (via drill 0.3)
  Top 0.406: R202.2 C204.1 68.57,85.09 v68.57,87
  Bottom 0.406: IC203.4 59.04,86.36 59.68,87 v68.57,87
N$27
  Top 0.406: D103.C 62.22,43.5 60.63,41.91 60.63,37.78 61.9,36.51 IC104.13
N$28  (via drill 0.3)
  Top 0.406: IC203.5 61.58,81.6 R202.1 v60.31,76.83 | IC202.11 IC202.12 | v58.09,72.07 58.09,76.52 v58.41,76.83
  Bottom 0.406: IC202.11 IC202.4 | IC202.12 51.74,70.8 53.01,72.07 v58.09,72.07 | v58.41,76.83 v60.31,76.83
N$29  (via drill 0.3)
  Top 0.406: IC104.12 IC104.11 | v58.09,31.43 57.77,31.11 R107.2 56.5,18.41 IC103.12
  Bottom 0.406: IC104.11 v58.09,31.43 IC104.4
N$30  (via drill 0.3)
  Top 0.406: IC202.13 52.06,73.34 52.38,73.03 v52.38,57.47
  Bottom 0.406: v52.38,57.47 63.17,57.47 D201.C
N$31
  Top 0.406: R107.1 C105.1
  Bottom 0.406: C105.1 47.61,17.46 48.25,18.1 53.64,18.1 53.96,17.78 IC103.13
N$32  (via drill 0.3)
  Top 0.406: v60.95,73.34 v60.95,53.02
  Bottom 0.406: IC204.13 v60.95,73.34 | v60.95,53.02 D202.C
N$33  (via drill 0.3)
  Top 0.406: IC104.8 v62.85,13.97 | v59.04,13.97 IC103.11
  Bottom 0.406: v62.85,13.97 v59.04,13.97
N$34  (via drill 0.3)
  Top 0.406: IC104.2 IC104.3 | v59.68,33.97 v59.68,28.89 59.68,21.91 60.31,21.27 R108.1 61.58,18.41 IC103.10
  Bottom 0.406: IC104.3 v59.68,33.97 | v59.68,28.89 IC104.10
N$35  (via drill 0.3)
  Top 0.406: IC203.12 56.5,89.53 57.77,88.27 R203.2 57.77,79.38 v56.18,77.79 | IC204.11 IC204.12 | v52.38,77.79 52.38,74.3 53.33,73.34 v53.33,68.26
  Bottom 0.406: IC204.11 IC204.4 v53.33,68.26 | v56.18,77.79 v52.38,77.79
N$36
  Top 0.406: R108.2 C106.1
  Bottom 0.406: IC103.9 64.12,17.46 64.76,18.1 68.88,18.1 R108.2
N$37  (via drill 0.3)
  Top 0.406: v66.66,30.16 IC103.8
  Bottom 0.406: IC104.5 56.82,28.89 58.09,30.16 v66.66,30.16
N$38
  Top 0.406: IC203.13 53.96,87.95 52.38,86.36 51.42,86.36 48.25,83.19 C205.1 R203.1
N$39  (via drill 0.3)
  Top 0.406: IC203.11 59.04,89.22 60.31,87.95 60.31,82.23 59.04,80.96 59.04,77.79 59.36,77.47 59.36,76.52 59.04,76.2 v59.04,60.64
  Bottom 0.406: v59.04,60.64 IC204.8
N$41  (via drill 0.3)
  Top 0.406: R204.1 61.58,93.34 IC203.10 61.58,89.22 62.85,87.95 v62.85,77.79 | v57.46,77.79 57.46,73.66 57.14,73.34 IC204.2 IC204.3 | v60,70.8 v60,65.72
  Bottom 0.406: v62.85,77.79 v57.46,77.79 | IC204.3 v60,70.8 | v60,65.72 IC204.10
N$42
  Bottom 0.406: OK301.3 R303.1
N$43
  Top 0.406: C206.1 R204.2 65.08,94.61 64.12,93.66 IC203.9
N$44  (via drill 0.3)
  Top 0.406: IC203.8 66.66,88.27 65.39,87 65.39,79.38 65.71,79.06 65.71,67.31 v66.03,66.99
  Bottom 0.406: v66.03,66.99 59.68,66.99 58.41,65.72 IC204.5
N$45  (via drill 0.3)
  Top 0.406: IC301.2 IC301.3 | v31.42,33.97 v31.42,28.89 31.42,18.1 31.74,17.78 31.74,11.11 30.47,9.84 IC302.2 30.47,6.35 31.42,5.4 R301.2
  Bottom 0.406: IC301.3 v31.42,33.97 | v31.42,28.89 IC301.10
N$46  (via drill 0.3)
  Top 0.406: X301.3 6.59,8.95 6.02,9.53 6.02,13.65 8.24,15.88 10.46,15.88 11.1,16.51 v11.1,58.74 | R304.2 19.67,61.28 20.94,60.01 OK301.1
  Bottom 0.406: v11.1,58.74 OK301.1
N$51
  Bottom 0.406: IC205.4 67.93,62.87 66.35,64.45 59.04,64.45 57.77,63.18 IC204.6
N$52  (via drill 0.3)
  Top 0.406: v60,72.07 v60,75.88
  Bottom 0.406: IC205.1 66.98,70.48 65.39,72.07 v60,72.07 | v60,75.88 IC204.1
N$53  (via drill 0.3)
  Top 0.406: v48.25,63.18 48.25,52.07 v48.88,51.44
  Bottom 0.406: IC202.6 v48.25,63.18 | v48.88,51.44 69.2,51.44 69.52,51.12 IC201.4
N$54  (via drill 0.3)
  Top 0.406: v47.29,58.74 v47.29,75.88
  Bottom 0.406: IC201.1 v47.29,58.74 | v47.29,75.88 IC202.1
N$55  (via drill 0.3)
  Top 0.406: R201.2 55.87,94.61 55.23,93.98 55.23,87 53.96,85.72 IC203.2 53.96,79.06 53.33,78.42 v53.33,74.61 | IC202.3 IC202.2 | v46.03,65.72 v46.03,70.8
  Bottom 0.406: v53.33,74.61 46.66,74.61 45.39,73.34 IC202.2 | IC202.10 v46.03,65.72 | v46.03,70.8 IC202.3
RXD
  Top 0.406: IC303.4 20.94,32.07 26.66,26.35 IC301.6
TRACK-0-E  (via drill 0.3)
  Top 1.016: X401.1 87.94,93.66 87.62,93.34 87.62,89.85 86.66,88.9 86.66,82.23 87.62,81.28 v87.62,78.42 v87.62,58.1 v87.62,37.78 v87.62,17.78
  Bottom 1.016: v87.62,17.78 90.86,17.78 X402.1 | X405.1 92.7,77.47 91.74,78.42 v87.62,78.42 | X404.1 92.7,57.15 91.74,58.1 v87.62,58.1 | X403.1 92.7,36.83 91.74,37.78 v87.62,37.78
TRACK-B-E
  Top 1.016: X402.2 89.52,14.92 89.21,15.24 89.21,35.24 | 89.21,35.24 89.21,55.56 | 89.21,55.56 89.21,75.88 | 89.21,75.88 89.21,87.95 89.84,88.58 X401.2 | X403.2 89.21,35.24 | X404.2 89.21,55.56 | X405.2 89.21,75.88
TXD
  Top 0.406: IC303.1 22.85,51.12 24.12,49.85 24.12,40.96 26.02,39.05 IC301.1
V-NETZTEIL
  Top 1.016: CON401.1 15.86,90.49 17.13,91.76 22.21,91.76 24.44,93.98 D401.A

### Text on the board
Bottom: (c) Dr.-Ing. Th. Wiesner | MBCAN-Projekt | 12.04.2024 | mbc_95_24_03_10.brd
tNames: HW: 24.03.10 | Zentrale | 0 | B | +18V | DC | Traffic | (c) Dr.-Ing. Th. Wiesner | MBCAN-Projekt | CAN D | CAN C | IN | CAN B | OUT | CAN A | mbc-95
